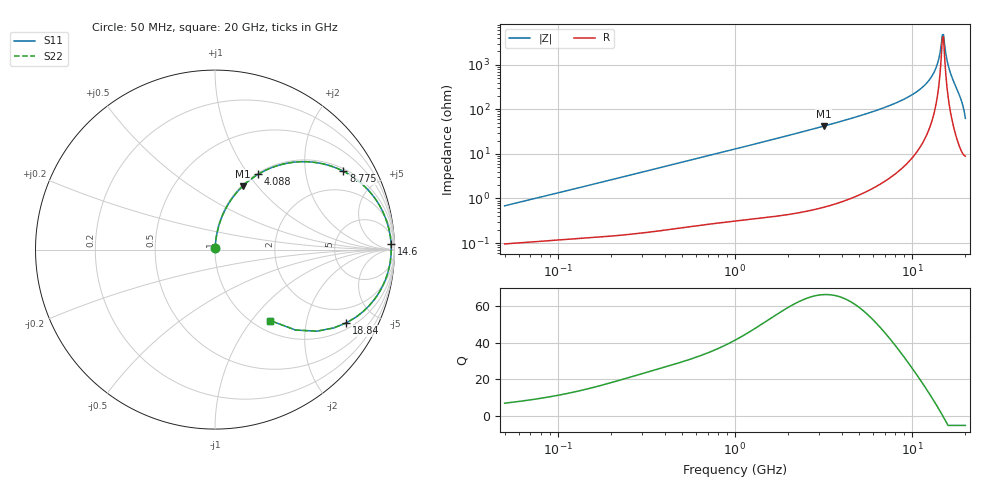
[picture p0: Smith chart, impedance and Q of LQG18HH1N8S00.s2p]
!Murata Part Number: LQG18HH1N8S00
!These Parameters are Measured in Series Mode Connection
!  o--[Z]--o
!Port1  Port2
!  o-------o
!Freq. Start=50[MHz] Stop=20[GHz], 401[Steps]
# Hz S RI R 50
!Freq.(Hz) S11(Real) S11(Imag) S21(Real) S21(Imag) S12(Real) S12(Imag) S22(Real) S22(Imag)
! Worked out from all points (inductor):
!   401 points, 50 MHz to 20 GHz, reference 50 ohm
!   read as one part in series: L = 2.14 nH near 51.52 MHz
!   highest Q = 66.2 at 3.169 GHz (marker M1), where L = 2.11 nH
!   self-resonance near 14.82 GHz
!   S11 on the Smith chart (normalised r, x): 50 MHz: 1.00, +0.01; 4.088 GHz: 1.02, +1.11; 8.775 GHz: 1.10, +3.21; 14.6 GHz: 29, +48; 18.84 GHz: 1.25, -3.42; 20 GHz: 1.18, -1.24
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5e7  0.001 0.00677  0.999 -0.00677  0.999 -0.00677  0.001 0.00677
1.364002e8  0.0016 0.018  0.9984 -0.018  0.9984 -0.018  0.0016 0.018
3.721004e8  0.0042 0.0482  0.9958 -0.0482  0.9958 -0.0482  0.0042 0.0482
1e9  0.0193 0.1259  0.9807 -0.1259  0.9807 -0.1259  0.0193 0.1259
2.728004e9  0.1173 0.3142  0.8827 -0.3142  0.8827 -0.3142  0.1173 0.3142
3.168813e9  0.1537 0.3532  0.8463 -0.3532  0.8463 -0.3532  0.1537 0.3532
4.087748e9  0.2399 0.4193  0.7601 -0.4193  0.7601 -0.4193  0.2399 0.4193
7.442007e9  0.592 0.4798  0.408 -0.4798  0.408 -0.4798  0.592 0.4798
8.774992e9  0.715 0.4368  0.285 -0.4368  0.285 -0.4368  0.715 0.4368
1.082228e10  0.8616 0.3228  0.1384 -0.3228  0.1384 -0.3228  0.8616 0.3228
1.257102e10  0.9416 0.1966  0.0584 -0.1966  0.0584 -0.1966  0.9416 0.1966
1.375312e10  0.9718 0.1018  0.0282 -0.1018  0.0282 -0.1018  0.9718 0.1018
1.417136e10  0.9777 0.0667  0.0223 -0.0667  0.0223 -0.0667  0.9777 0.0667
1.460232e10  0.9811 0.0298  0.0189 -0.0298  0.0189 -0.0298  0.9811 0.0298
1.482269e10  0.9818 0.0106  0.0182 -0.0106  0.0182 -0.0106  0.9818 0.0106
1.504638e10  0.9817 -0.00923  0.0183 0.00923  0.0183 0.00923  0.9817 -0.00923
1.527346e10  0.9807 -0.0296  0.0193 0.0296  0.0193 0.0296  0.9807 -0.0296
1.597544e10  0.9715 -0.0947  0.0285 0.0947  0.0285 0.0947  0.9715 -0.0947
1.646126e10  0.9588 -0.1421  0.0412 0.1421  0.0412 0.1421  0.9588 -0.1421
1.774144e10  0.8869 -0.2794  0.1131 0.2794  0.1131 0.2794  0.8869 -0.2794
1.88369e10  0.7313 -0.4084  0.2687 0.4084  0.2687 0.4084  0.7313 -0.4084
2e10  0.3071 -0.3951  0.6929 0.3951  0.6929 0.3951  0.3071 -0.3951
